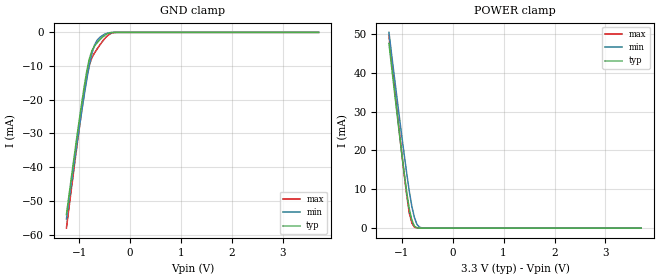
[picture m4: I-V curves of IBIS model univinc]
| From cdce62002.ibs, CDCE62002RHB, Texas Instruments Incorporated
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|   Model   univinc
[Model]   univinc
Model_type   Input
Polarity   Non-Inverting
Vinl   =   0.99V
Vinh   =   2.31V
|Variable   typ   min   max
C_comp   9.336e-13   8.788e-13   2.334e-12
[Model Spec]
Vinl   0.99V   0.9V   1.08V
Vinh   2.31V   2.1V   2.52V
|Variable   typ   min   max
[Voltage range]   3.3   3.0   3.6
|Variable   typ   min   max
[Temperature range]  25   85   0
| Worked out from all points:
|   GND clamp passes 1 mA (typ) near -0.51 V on its own axis
|   POWER clamp passes 1 mA (typ) near -0.77 V on its own axis
[GND_clamp]
|Volts   typ   min   max
-1.25V    -54.09mA   -55.39mA   -58.09mA
-1.1V     -37.11mA   -39.01mA   -40.22mA
-950mV    -20.95mA   -23.44mA   -23.18mA
-850mV    -11.46mA   -13.91mA   -13.26mA
-800mV    -7.838mA   -9.726mA   -9.695mA
-750mV    -5.437mA   -6.264mA   -7.495mA
-700mV    -4.095mA   -3.791mA   -6.14mA
-650mV    -3.122mA   -2.379mA   -4.981mA
-550mV    -1.519mA   -976.4uA   -2.813mA
-400mV    -148uA     -91.99uA   -478.2uA
-250mV    -1.556uA   -1.907uA   -5.69uA
3.7V      0A         0A         0A
[POWER_clamp]
|Volts   typ   min   max
-1.25V    47.56mA    50.37mA    49.63mA
-1.05V    24.87mA    29.06mA    25.31mA
-950mV    14.13mA    18.87mA    13.77mA
-900mV    9.116mA    14.02mA    8.406mA
-850mV    4.865mA    9.437mA    3.87mA
-800mV    2.05mA     5.557mA    1.329mA
-750mV    528.7uA    2.738mA    250.1uA
-700mV    89.03uA    963.7uA    32.78uA
-650mV    13.1uA     241.3uA    3.97uA
-550mV    271.4nA    10.2uA     59.49nA
3.7V      0A         0A         0A
